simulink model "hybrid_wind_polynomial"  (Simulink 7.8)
settings: Solver=FixedStepDiscrete  SolverMode=SingleTasking  StartTime=0.0  StopTime=runtime  FixedStep=Ts  RelTol=1e-3
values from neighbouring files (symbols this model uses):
  alpha = 0.5    [bowed_string_hyperbolic.m]    (also in polynomial.m = 100)
  amp_gain_factor = 0.73316    [hybrid_wind.m]    (also in measurements.m = 0.73312)
  delta_cte = 0.1    [polynomial.m]
  HLL_d = c2d(HLL_c,Ts)    [hybrid_wind.m]    (also in measurements.m)
  maxoutputvoltage = 5    [hybrid_wind.m]    (also in measurements.m)
  micoffset_V = mean(voltsin_calib)    [hybrid_wind.m]    (also in measurements.m)
  micpreampsensitivity = -0.0025726    [hybrid_wind.m]    (also in measurements.m)
  Ts = 25e-6    (= 2.5e-05)    [hybrid_wind.m]    (also in measurements.m)
  Zc = rho*c/St    (= 2615281.00417)    [hybrid_wind.m]
  zeta_cte = 0.08    [polynomial.m]
undefined symbols (not defined in the file or in its folder): Bl, cell2mat, Mms, Re, Sd, vibrato
libraries: simulink x2

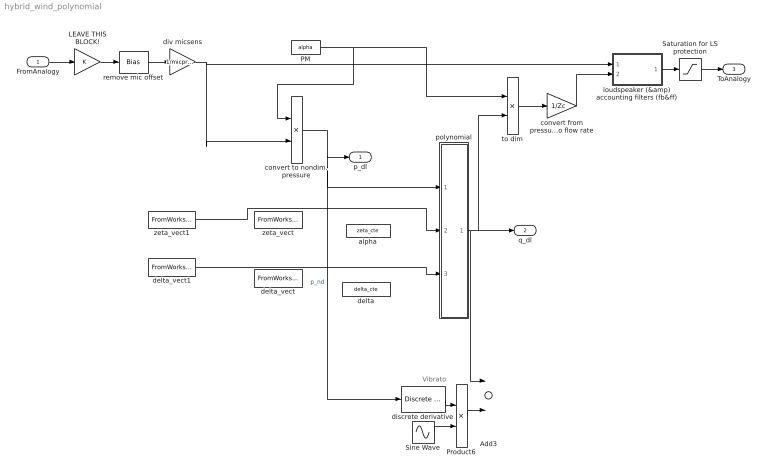
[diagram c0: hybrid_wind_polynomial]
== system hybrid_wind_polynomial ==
  note: Vibrato
  FromAnalogy : Inport  Interpolate=off
  Add3 : Sum
  LEAVE THIS BLOCK! : Gain
  PM : Constant  Value=alpha
  Product6 : Product
  Saturation for LS protection : Saturate  UpperLimit=maxoutputvoltage  LowerLimit=-maxoutputvoltage
  Sine Wave : Sin  Amplitude=vibrato.amp  Bias=-vibrato.amp  Frequency=vibrato.freq*2*pi  SampleTime=0
  alpha : Constant  Value=zeta_cte
  convert from pressure  to flow rate : Gain  Gain=1/Zc
  convert to nondim. pressure : Product  Inputs=/*
  delta : Constant  Value=delta_cte
  delta_vect : FromWorkspace  VariableName=delta_vect  SampleTime=Ts  OutputAfterFinalValue=Setting to zero
  delta_vect1 : FromWorkspace  VariableName=delta_envs_all  SampleTime=Ts  OutputAfterFinalValue=Setting to zero
  discrete derivative : simulink/Discrete/Discrete Derivative  gainval=1.0  ICPrevScaledInput=0.0  InputProcessing=Inherited  OutMin=[]  OutMax=[]  OutDataType=fixdt(1, 16)  OutScaling=2^-10  DoSatur=off
  div micsens : Gain  Gain=1/micpreampsensitivity
  loudspeaker (&amp) accounting filters (fb&ff) : Subsystem
  polynomial : Subsystem
  remove mic offset : Bias  Bias=-micoffset_V
  to dim : Product
  zeta_vect : FromWorkspace  VariableName=zeta_vect  SampleTime=Ts  OutputAfterFinalValue=Setting to zero
  zeta_vect1 : FromWorkspace  VariableName=zeta_envs_all  SampleTime=Ts  OutputAfterFinalValue=Setting to zero
  p_dl : Outport
  q_dl : Outport  Port=2
  ToAnalogy : Outport  Port=3
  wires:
  convert to nondim. pressure/1 -> p_dl/1, polynomial/1(pdl), discrete derivative/1  "p_nd"
  div micsens/1 -> loudspeaker (&amp) accounting filters (fb&ff)/1(P), convert to nondim. pressure/2
  FromAnalogy/1 -> LEAVE THIS BLOCK!/1
  Saturation for LS protection/1 -> ToAnalogy/1
  loudspeaker (&amp) accounting filters (fb&ff)/1(V_amp_in) -> Saturation for LS protection/1
  to dim/1 -> convert from pressure  to flow rate/1
  convert from pressure  to flow rate/1 -> loudspeaker (&amp) accounting filters (fb&ff)/2(Q_calc)
  discrete derivative/1 -> Product6/1
  Sine Wave/1 -> Product6/2
  Product6/1 -> Add3/2
  polynomial/1(qdl) -> to dim/2, q_dl/1, Add3/1
  Add3/1 -> ?  "new fdl"
  remove mic offset/1 -> div micsens/1
  LEAVE THIS BLOCK!/1 -> remove mic offset/1
  PM/1 -> to dim/1, convert to nondim. pressure/1
  zeta_vect1/1 -> polynomial/2(zeta)
  delta_vect1/1 -> polynomial/3(delta)

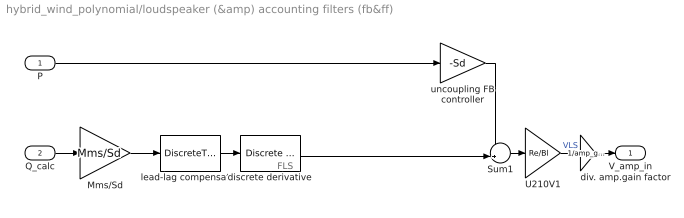
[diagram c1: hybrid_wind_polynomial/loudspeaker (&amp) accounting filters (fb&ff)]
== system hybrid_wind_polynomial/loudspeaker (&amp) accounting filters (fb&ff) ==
  note: FLS
  P : Inport
  Q_calc : Inport  Port=2
  Mms/Sd : Gain  Gain=Mms/Sd
  Sum1 : Sum  Inputs=-+|
  U210V1 : Gain  Gain=Re/Bl
  discrete derivative : simulink/Discrete/Discrete Derivative  gainval=1.0  ICPrevScaledInput=0.0  InputProcessing=Inherited  OutMin=[]  OutMax=[]  OutDataType=fixdt(1, 16)  OutScaling=2^-10  DoSatur=off
  div. amp.gain factor : Gain  Gain=1/amp_gain_factor
  lead-lag compensator : DiscreteTransferFcn  Numerator=cell2mat(HLL_d.num)  Denominator=cell2mat(HLL_d.den)  SampleTime=Ts
  uncoupling FB controller : Gain  Gain=-Sd
  V_amp_in : Outport
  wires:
  Sum1/1 -> U210V1/1
  U210V1/1 -> div. amp.gain factor/1  "VLS"
  Q_calc/1 -> Mms/Sd/1
  discrete derivative/1 -> Sum1/2
  uncoupling FB controller/1 -> Sum1/1
  div. amp.gain factor/1 -> V_amp_in/1
  P/1 -> uncoupling FB controller/1
  Mms/Sd/1 -> lead-lag compensator/1
  lead-lag compensator/1 -> discrete derivative/1

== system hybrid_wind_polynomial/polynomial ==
  pdl : Inport
  zeta : Inport  Port=2
  delta : Inport  Port=3
  Add3 : Sum  Inputs=-+
  Unit Delay : UnitDelay  SampleTime=-1
  calc. real root of 3rd order eq ->old! : Subsystem
  implicit to explicit + calc real root of 3rd order eq. : S-Function  InitFcn=try, set_param(gcb,'FunctionName','polynomial_excitation'), end  FunctionName=polynomial_excitation  SFunctionModules=polynomial_excitation_wrapper  WizardData=DataTag0  EnableBusSupport=off
  qdl : Outport
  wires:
  zeta/1 -> implicit to explicit + calc real root of 3rd order eq./2
  delta/1 -> implicit to explicit + calc real root of 3rd order eq./3
  implicit to explicit + calc real root of 3rd order eq./1 -> Unit Delay/1, qdl/1
  pdl/1 -> Add3/2
  Unit Delay/1 -> Add3/1  "approximative q[n]"
  Add3/1 -> implicit to explicit + calc real root of 3rd order eq./1  "pretneding to be phdl but is actually phdl\u001dn-1"

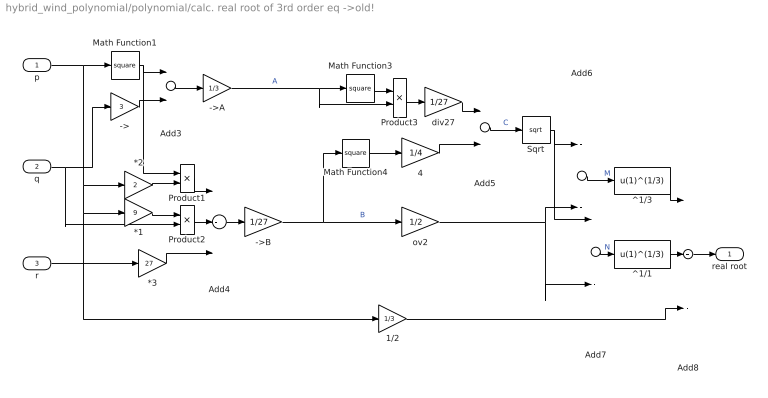
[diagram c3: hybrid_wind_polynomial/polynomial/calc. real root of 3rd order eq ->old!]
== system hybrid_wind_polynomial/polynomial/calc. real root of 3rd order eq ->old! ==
  p : Inport
  q : Inport  Port=2
  r : Inport  Port=3
  *1 : Gain  Gain=9
  *2 : Gain  Gain=2
  *3 : Gain  Gain=27
  -> : Gain  Gain=3
  ->A : Gain  Gain=1/3
  ->B : Gain  Gain=1/27
  1/2 : Gain  Gain=1/3
  4 : Gain  Gain=1/4
  Add3 : Sum  Inputs=-+
  Add4 : Sum  Inputs=+-+
  Add5 : Sum
  Add6 : Sum  Inputs=+-
  Add7 : Sum  Inputs=--
  Add8 : Sum  Inputs=++-
  Math Function1 : Math  Operator=square
  Math Function3 : Math  Operator=square
  Math Function4 : Math  Operator=square
  Product1 : Product
  Product2 : Product
  Product3 : Product
  Sqrt : Sqrt
  ^1/1 : Fcn  Expr=u(1)^(1/3)
  ^1/3 : Fcn  Expr=u(1)^(1/3)
  div27 : Gain  Gain=1/27
  ov2 : Gain  Gain=1/2
  real root : Outport
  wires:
  p/1 -> 1/2/1, *1/1, *2/1, Math Function1/1
  q/1 -> Product2/2, ->/1
  Math Function1/1 -> Add3/1, Product1/1
  ->/1 -> Add3/2
  Add3/1 -> ->A/1
  ->A/1 -> Math Function3/1, Product3/2  "A"
  Product1/1 -> Add4/1
  Add4/1 -> ->B/1
  ->B/1 -> Math Function4/1, ov2/1  "B"
  *2/1 -> Product1/2
  Product2/1 -> Add4/2
  *1/1 -> Product2/1
  *3/1 -> Add4/3
  Math Function3/1 -> Product3/1
  Product3/1 -> div27/1
  div27/1 -> Add5/1
  Math Function4/1 -> 4/1
  4/1 -> Add5/2
  Add5/1 -> Sqrt/1  "C"
  Sqrt/1 -> Add6/1, Add7/1
  ov2/1 -> Add6/2, Add7/2
  1/2/1 -> Add8/3
  Add6/1 -> ^1/3/1  "M"
  ^1/3/1 -> Add8/1
  Add7/1 -> ^1/1/1  "N"
  ^1/1/1 -> Add8/2
  Add8/1 -> real root/1
  r/1 -> *3/1
